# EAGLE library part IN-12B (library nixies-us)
IN-12B: medium numeric topview nixie tube
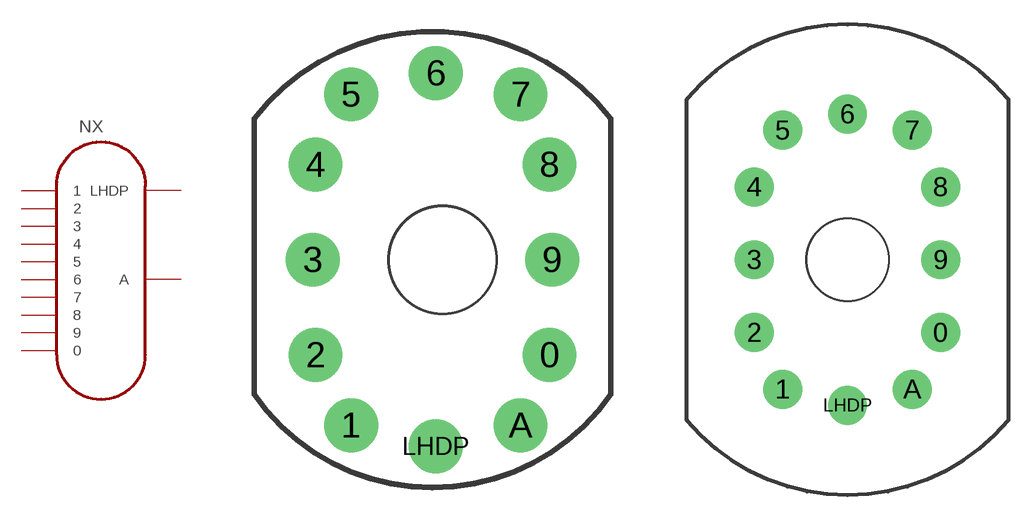
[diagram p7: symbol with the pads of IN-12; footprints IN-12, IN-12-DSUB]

Designator prefix NX

## IN-12BORIGINAL  [IN-12]
0  0
1  1
2  2
3  3
4  4
5  5
6  6
7  7
8  8
9  9
A  A
LHDP  LHDP

## IN-12BIN-12-DSUB  [IN-12-DSUB]
Pads as for IN-12

## IN-12BNOHOLE  [IN-12-DSUB-NOHOLE]
Pads as for IN-12

## Footprint IN-12 (pad centres in mm)
May be used with socket: SK-136
drill 1.1 pad 2.54: 0 5.048,-4.5; 1 -4.317,-7.817; 2 -6,-4.5; 3 -6.127,0; 4 -6,4.5; 5 -4.317,7.817; 6 -0.318,8.818; 7 3.683,7.817; 8 5.048,4.5; 9 5.175,0; A 3.683,-7.817; LHDP -0.318,-8.818
hole 5 at 0,0

## Footprint IN-12-DSUB (pad centres in mm)
For use with female D-SUB pins
drill 1.6: 0 5.75,-4.5; 1 -4,-8; 2 -5.75,-4.5; 3 -5.75,0; 4 -5.75,4.5; 5 -4,8; 6 0,9; 7 4,8; 8 5.75,4.5; 9 5.75,0; A 4,-8; LHDP 0,-9
hole 5 at 0,0

## Footprint IN-12-DSUB-NOHOLE (pad centres in mm)
For use with female D-SUB pins
drill 1.6: 0 5.75,-4.5; 1 -4,-8; 2 -5.75,-4.5; 3 -5.75,0; 4 -5.75,4.5; 5 -4,8; 6 0,9; 7 4,8; 8 5.75,4.5; 9 5.75,0; A 4,-8; LHDP 0,-9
